| TEXAS INSTRUMENTS INCORPORATED
| Standard Linear and Logic Group
| IBIS Model of TS3A5018
| 10 Ohm Quad SPDT Analog Switch
| This file contains package information for the following:
|  SOIC 16-pin (D) package as [Component] TS3A5018_D
|  SSOP 16-pin (DBQ) package as [Component] TS3A5018_DBQ
|  TVSOP 16-pin (DGV) package as [Component] TS3A5018_DGV
|  TSSOP 16-pin (PW) package as [Component] TS3A5018_PW
| This device can be powered at the following Vccs:
|  3.3 volt Vcc
|  2.5 volt Vcc
| This file provides unique models under the [Model Selector] for each Vcc.
| For operation at a specific Vcc, select the appropriate model after each
| [Model Selector] keyword.
[IBIS Ver]   3.2
[Comment char]  |_char
[File Name]   ts3a5018.ibs
[File Rev]   1.1 | a_die
[Date]   January 25, 2007
[Source]   Data created from TI-SPICE simulations at TI-SLL.
[Notes]   The following is an IBIS list for the TS3A5018.
   Please contact sllibis@ti.com with questions and
   comments concerning SLL IBIS models.
   - FILE REV HISTORY
   - 1.1 Release IBIS file on 05/23/08
   - Power clamp data deleted was deleted as there is no
   power-clamp diode.
   - Non-monotonic data due to FET characteristics.
[Disclaimer] Property of Texas Instruments Incorporated.  Unauthorized
   reproduction and/or distribution is strictly prohibited.
   This product is protected under copyright law.
   Created  2007, (C) Copyright  2007, Texas Instruments
   Incorporated, All Rights Reserved
   UNLESS THERE IS A SIGNED, WRITTEN AGREEMENT TO THE
   CONTRARY, TEXAS INSTRUMENTS (TI) IS PROVIDING THE IBIS
   MODELS  AND WITHOUT ANY WARRANTY, EXPRESSED OR
   IMPLIED.  TI assumes no liability for:
   1) the accuracy of the IBIS models provided to your
   company;
   2) the proper functioning of these IBIS Models in your
   design or for any resulting applications; or
   3) infringement of patents, copyrights or intellectual
   property rights resulting from your use of these IBIS
   models.
   TI provides IBIS Models as a service to our customers.
   You and your company shall not distribute, sell or give
   these models to anyone else without prior written
   permission from TI.
   TI reserves the right to make changes to our products or
   to discontinue any semiconductor product or service
   without notice, and advises our customers to obtain the
   latest version of relevant information to verify, before
   placing orders, that the information being relied on is
   current.
   Please be aware that your receipt and use of the IBIS
   information provided shall serve as acceptance of these
   terms and conditions.  If you do not accept these terms,
   you should return or destroy the IBIS models and any
   other accompanying information immediately.
| Component TS3A5018_D 16-PIN SOIC
[Component]   TS3A5018_D
[Manufacturer]   Texas Instruments, Inc.
[Package]
|   typ   min   max
R_pkg   3.900e-02   2.800e-02   4.900e-02
L_pkg   3.453e-09   2.350e-09   4.375e-09
C_pkg   5.210e-13   2.540e-13   7.080e-13
[Pin]   signal_name   model_name   R_pin   L_pin   C_pin
1   IN   TS3A5018_IN   4.200e-02   4.336e-09   7.030e-13
2   NC1   TS3A5018_NX   4.900e-02   3.778e-09   6.340e-13
3   NO1   TS3A5018_NX   2.800e-02   3.449e-09   5.180e-13
4   COM1   TS3A5018_COM   2.900e-02   2.393e-09   2.540e-13
5   NC2   TS3A5018_NX   2.800e-02   2.350e-09   2.640e-13
6   NO2   TS3A5018_NX   4.800e-02   3.312e-09   4.830e-13
7   COM2   TS3A5018_COM   4.300e-02   3.629e-09   6.040e-13
8   GND   GND   4.400e-02   4.375e-09   7.080e-13
9   COM3   TS3A5018_COM   4.200e-02   4.336e-09   7.030e-13
10   NO3   TS3A5018_NX   4.900e-02   3.778e-09   6.340e-13
11   NC3   TS3A5018_NX   2.800e-02   3.449e-09   5.180e-13
12   COM4   TS3A5018_COM   2.900e-02   2.393e-09   2.550e-13
13   NO4   TS3A5018_NX   2.800e-02   2.350e-09   2.640e-13
14   NC4   TS3A5018_NX   4.800e-02   3.312e-09   4.830e-13
15   NOE   TS3A5018_IN   4.300e-02   3.629e-09   6.040e-13
16   VCC   POWER   4.400e-02   4.375e-09   7.080e-13
| Component TS3A5018_DBQ 16-PIN SSOP
[Component]   TS3A5018_DBQ
[Manufacturer]   Texas Instruments, Inc.
[Package]
|   typ   min   max
R_pkg   3.800e-02   2.700e-02   5.900e-02
L_pkg   2.353e-09   1.491e-09   4.500e-09
C_pkg   2.100e-13   6.400e-14   5.920e-13
[Pin]   signal_name   model_name   R_pin   L_pin   C_pin
1   IN   TS3A5018_IN   5.800e-02   4.450e-09   5.920e-13
2   NC1   TS3A5018_NX   4.000e-02   1.930e-09   1.110e-13
3   NO1   TS3A5018_NX   2.800e-02   1.538e-09   7.600e-14
4   COM1   TS3A5018_COM   2.700e-02   1.491e-09   6.400e-14
5   NC2   TS3A5018_NX   2.700e-02   1.491e-09   6.400e-14
6   NO2   TS3A5018_NX   2.700e-02   1.506e-09   7.500e-14
7   COM2   TS3A5018_COM   3.300e-02   1.922e-09   1.090e-13
8   GND   GND   5.900e-02   4.500e-09   5.880e-13
9   COM3   TS3A5018_COM   5.800e-02   3.695e-09   4.140e-13
10   NO3   TS3A5018_NX   3.400e-02   2.685e-09   2.820e-13
11   NC3   TS3A5018_NX   2.900e-02   1.552e-09   7.700e-14
12   COM4   TS3A5018_COM   2.800e-02   1.506e-09   6.500e-14
13   NO4   TS3A5018_NX   2.700e-02   1.492e-09   6.400e-14
14   NC4   TS3A5018_NX   2.800e-02   1.534e-09   7.600e-14
15   NOE   TS3A5018_IN   4.000e-02   2.703e-09   2.840e-13
16   VCC   POWER   5.600e-02   3.645e-09   4.180e-13
| Component TS3A5018_DGV 16-pin TVSOP
[Component]   TS3A5018_DGV
[Manufacturer]   Texas Instruments, Inc.
[Package]
|   typ   min   max
R_pkg   3.900e-02   3.300e-02   4.500e-02
L_pkg   2.543e-09   2.320e-09   2.938e-09
C_pkg   3.860e-13   3.340e-13   4.490e-13
[Pin]   signal_name   model_name   R_pin   L_pin   C_pin
1   IN   TS3A5018_IN   3.500e-02   2.907e-09   4.170e-13
2   NC1   TS3A5018_NX   4.200e-02   2.558e-09   4.460e-13
3   NO1   TS3A5018_NX   3.800e-02   2.341e-09   3.450e-13
4   COM1   TS3A5018_COM   3.800e-02   2.320e-09   3.340e-13
5   NC2   TS3A5018_NX   3.900e-02   2.322e-09   3.340e-13
6   NO2   TS3A5018_NX   3.800e-02   2.353e-09   3.420e-13
7   COM2   TS3A5018_COM   4.000e-02   2.536e-09   4.410e-13
8   GND   GND   3.300e-02   2.897e-09   4.180e-13
9   COM3   TS3A5018_COM   3.500e-02   2.927e-09   4.190e-13
10   NO3   TS3A5018_NX   4.500e-02   2.632e-09   4.490e-13
11   NC3   TS3A5018_NX   3.900e-02   2.368e-09   3.470e-13
12   COM4   TS3A5018_COM   3.900e-02   2.330e-09   3.350e-13
13   NO4   TS3A5018_NX   3.900e-02   2.320e-09   3.350e-13
14   NC4   TS3A5018_NX   3.900e-02   2.361e-09   3.450e-13
15   NOE   TS3A5018_IN   4.100e-02   2.573e-09   4.460e-13
16   VCC   POWER   3.500e-02   2.938e-09   4.200e-13
| Component TS3A5018_PW 16-PIN TSSOP
[Component]   TS3A5018_PW
[Manufacturer]   Texas Instruments, Inc.
[Package]
|   typ   min   max
R_pkg   4.500e-02   3.800e-02   5.100e-02
L_pkg   2.593e-09   2.447e-09   3.080e-09
C_pkg   2.810e-13   2.430e-13   3.770e-13
[Pin]   signal_name   model_name   R_pin   L_pin   C_pin
1   IN   TS3A5018_IN   4.000e-02   3.080e-09   3.770e-13
2   NC1   TS3A5018_NX   3.800e-02   2.458e-09   2.810e-13
3   NO1   TS3A5018_NX   5.100e-02   2.512e-09   2.550e-13
4   COM1   TS3A5018_COM   5.100e-02   2.447e-09   2.430e-13
5   NC2   TS3A5018_NX   5.100e-02   2.447e-09   2.430e-13
6   NO2   TS3A5018_NX   5.100e-02   2.512e-09   2.550e-13
7   COM2   TS3A5018_COM   3.800e-02   2.458e-09   2.810e-13
8   GND   GND   4.000e-02   3.080e-09   3.770e-13
9   COM3   TS3A5018_COM   3.900e-02   2.832e-09   3.160e-13
10   NO3   TS3A5018_NX   3.800e-02   2.460e-09   2.790e-13
11   NC3   TS3A5018_NX   5.100e-02   2.512e-09   2.550e-13
12   COM4   TS3A5018_COM   5.100e-02   2.447e-09   2.430e-13
13   NO4   TS3A5018_NX   5.100e-02   2.447e-09   2.430e-13
14   NC4   TS3A5018_NX   5.100e-02   2.512e-09   2.550e-13
15   NOE   TS3A5018_IN   3.800e-02   2.459e-09   2.790e-13
16   VCC   POWER   3.900e-02   2.832e-09   3.160e-13
[Series Switch Groups]
| Function Group States
On  1 /   | NC1-NC4->COM1-COM4 IN LOW
On  2 /   | NO1-NO4->COM1-COM4 IN HIGH
On  3 /   | COM1-COM4->NC1-NC4 IN LOW
On  4 /   | COM1-COM4->NO1-NO4 IN HIGH
On  1 2 3 4 /   | NOE LOW
Off 1 2 3 4 /   | NOE HIGH
[Series Pin Mapping]   pin_2   model_name   function_table_group
2   4   TS3A5018_NX_33_S   1
| 2   4   TS3A5018_NX_25_S   1
5   7   TS3A5018_NX_33_S   1
| 5   7   TS3A5018_NX_25_S   1
11   9   TS3A5018_NX_33_S   1
| 11   9   TS3A5018_NX_25_S   1
14   12   TS3A5018_NX_33_S   1
| 14   12   TS3A5018_NX_25_S   1
3   4   TS3A5018_NX_33_S   2
| 3   4   TS3A5018_NX_25_S   2
6   7   TS3A5018_NX_33_S   2
| 6   7   TS3A5018_NX_25_S   2
10   9   TS3A5018_NX_33_S   2
| 10   9   TS3A5018_NX_25_S   2
13   12   TS3A5018_NX_33_S   2
| 13   12   TS3A5018_NX_25_S   2
4   2   TS3A5018_COM_33_S   3
| 4   2   TS3A5018_COM_25_S   3
7   5   TS3A5018_COM_33_S   3
| 7   5   TS3A5018_COM_25_S   3
9   11   TS3A5018_COM_33_S   3
| 9   11   TS3A5018_COM_25_S   3
12   14   TS3A5018_COM_33_S   3
| 12   14   TS3A5018_COM_25_S   3
4   3   TS3A5018_COM_33_S   4
| 4   3   TS3A5018_COM_25_S   4
7   6   TS3A5018_COM_33_S   4
| 7   6   TS3A5018_COM_25_S   4
9   10   TS3A5018_COM_33_S   4
| 9   10   TS3A5018_COM_25_S   4
12   13   TS3A5018_COM_33_S   4
| 12   13   TS3A5018_COM_25_S   4
| Model TS3A5018_IN
[Model Selector]   TS3A5018_IN
TS3A5018_IN_33   3.3 volt Vcc
TS3A5018_IN_25   2.5 volt Vcc
| Model TS3A5018_NX
[Model Selector]   TS3A5018_NX
TS3A5018_NX_33   3.3 volt Vcc
TS3A5018_NX_25   2.5 volt Vcc
| Model TS3A5018_NX_S
[Model Selector]   TS3A5018_NX_S
TS3A5018_NX_33_S   3.3 volt Vcc
TS3A5018_NX_25_S   2.5 volt Vcc
| Model TS3A5018_COM
[Model Selector]   TS3A5018_COM
TS3A5018_COM_33   3.3 volt Vcc
TS3A5018_COM_25   2.5 volt Vcc
| Model TS3A5018_COM_S
[Model Selector]   TS3A5018_COM_S
TS3A5018_COM_33_S   3.3 volt Vcc
TS3A5018_COM_25_S   2.5 volt Vcc
[Model]   TS3A5018_NX_33_S
Model_type  Series_switch
| variable   typ   min   max
C_comp   0   0   0
[Temperature Range]   40   100   -40
| Ambient temperature   25   85   -40
[Voltage range]   3.3   3   3.6
[On]
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[Off]
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[Model]   TS3A5018_NX_25_S
Model_type  Series_switch
| variable   typ   min   max
C_comp   0   0   0
[Temperature Range]   40   100   -40
| Ambient temperature   25   85   -40
[Voltage range]   2.5   2.3   2.7
[On]
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[Off]
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[Model]   TS3A5018_COM_33_S
Model_type  Series_switch
| variable   typ   min   max
C_comp   0   0   0
[Temperature Range]   40   100   -40
| Ambient temperature   25   85   -40
[Voltage range]   3.3   3   3.6
[On]
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[Off]
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[Model]   TS3A5018_COM_25_S
Model_type  Series_switch
| variable   typ   min   max
C_comp   0   0   0
[Temperature Range]   40   100   -40
| Ambient temperature   25   85   -40
[Voltage range]   2.5   2.3   2.7
[On]
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[Off]
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| Models and submodels in the file (10): TS3A5018_IN_33 (Input), TS3A5018_IN_25 (Input), TS3A5018_NX_33_S (Series_switch), TS3A5018_NX_33 (Terminator), TS3A5018_NX_25_S (Series_switch), TS3A5018_NX_25 (Terminator), TS3A5018_COM_33_S (Series_switch), TS3A5018_COM_33 (Terminator), TS3A5018_COM_25_S (Series_switch), TS3A5018_COM_25 (Terminator)
